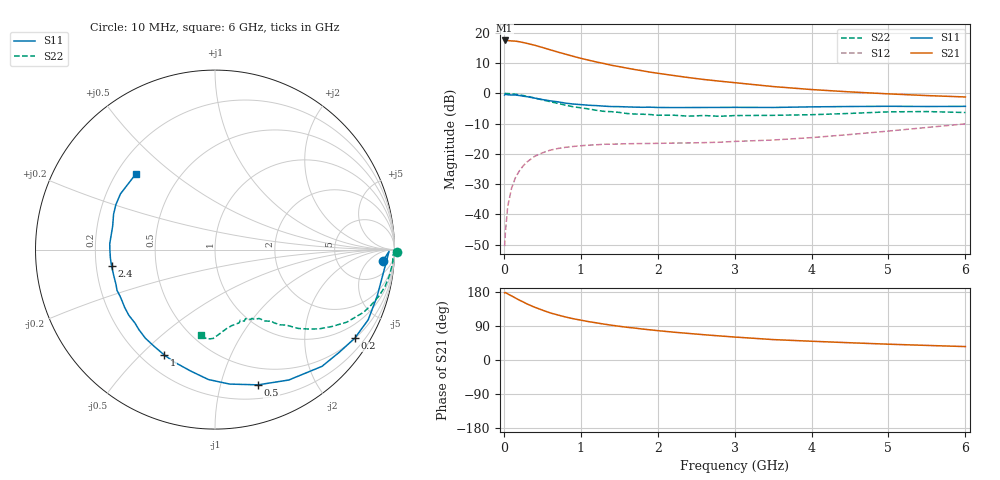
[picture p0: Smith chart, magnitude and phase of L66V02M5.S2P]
!  INFINEON TECHNOLOGIES Small Signal Semiconductors
! BFR380L3 , Si-NPN RF-Transistor in TSLP-3-1
!  Vce=6 V,  Ic=2.5 mA
! Common Emitter S-Parameters:  07. March 2005
#  GHz  S  MA  R  50
! f  S11  S21  S12  S22
! GHz  Mag  Ang  Mag  Ang  Mag  Ang  Mag  Ang
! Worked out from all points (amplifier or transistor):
!   36 points, 10 MHz to 6 GHz, reference 50 ohm
!   highest |S21| = 17.5 dB at 10 MHz (marker M1)
!   |S21| within 3 dB of that: start of sweep to 591.5 MHz
!   unconditionally stable (mu >= 1): 3.129 GHz to 4.479 GHz
!   at 250 MHz: K = 0.09, MSG = 20.4 dB, |S12| = -24.0 dB
!   at 1.4 GHz: K = 0.56, MSG = 13.0 dB, |S12| = -16.8 dB
!   at 6 GHz: K = 0.88, MSG = 4.4 dB, |S12| = -10.1 dB
!   S11 on the Smith chart (normalised r, x): 10 MHz: 14, -15; 200 MHz: 0.51, -3.37; 500 MHz: 0.33, -1.31; 1 GHz: 0.29, -0.59; 2.4 GHz: 0.26, -0.07; 6 GHz: 0.28, +0.38
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0.01  0.9359 -4.0  7.47 177.2  0.003 83.7  1.015 -0.9
0.02  0.9698 -0.6  7.435 178.1  0.005 91.6  0.9919 -1.7
0.05  0.946 -8.3  7.435 174.5  0.0135 87.0  0.9931 -4.1
0.1  0.94 -16.0  7.344 169.2  0.0271 81.1  0.9833 -8.2
0.15  0.939 -24.6  7.283 163.7  0.0404 75.9  0.9692 -12.3
0.2  0.9218 -32.4  7.119 158.1  0.0521 73.1  0.9495 -15.8
0.3  0.8823 -47.5  6.687 148.1  0.0735 65.2  0.8984 -22.9
0.4  0.8348 -60.5  6.229 139.3  0.0913 58.5  0.8386 -28.8
0.5  0.7905 -72.4  5.729 131.7  0.1041 53.2  0.7813 -33.2
0.6  0.7536 -83.8  5.249 124.5  0.1151 48.5  0.7303 -37.2
0.7  0.7249 -92.9  4.815 118.9  0.1228 45.3  0.6827 -40.4
0.9  0.6665 -109.8  4.094 109.0  0.1327 39.6  0.6005 -45.4
1  0.6519 -115.6  3.791 105.2  0.1364 38.5  0.5779 -46.7
1.1  0.6367 -122.2  3.536 101.3  0.1397 36.7  0.5535 -49.2
1.3  0.6154 -133.5  3.112 94.8  0.1444 35.0  0.5048 -51.9
1.6  0.5976 -147.4  2.61 86.4  0.1474 33.7  0.4646 -56.6
2.2  0.5824 -165.8  1.976 73.6  0.1512 36.1  0.4363 -63.0
2.4  0.5833 -170.9  1.823 70.1  0.1518 37.7  0.4206 -66.2
3.5  0.5849 167.1  1.295 53.9  0.1696 48.4  0.4336 -77.5
4.5  0.6065 155.6  1.057 45.5  0.2093 59.0  0.4664 -86.2
5.5  0.6069 143.3  0.919 38.5  0.2734 63.7  0.5006 -95.0
6  0.61 136.1  0.872 35.4  0.3135 63.7  0.4828 -99.3
